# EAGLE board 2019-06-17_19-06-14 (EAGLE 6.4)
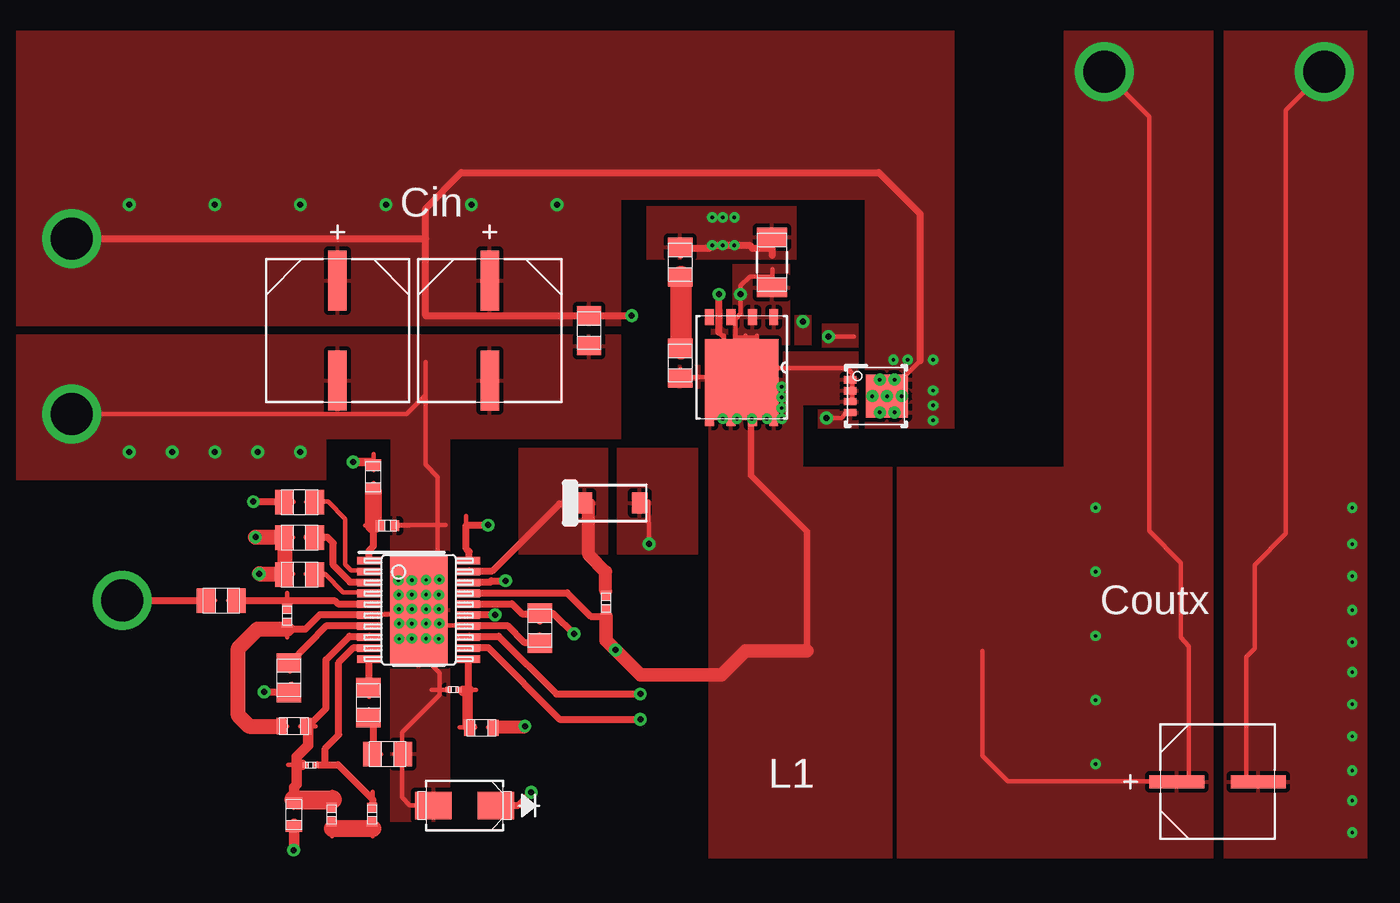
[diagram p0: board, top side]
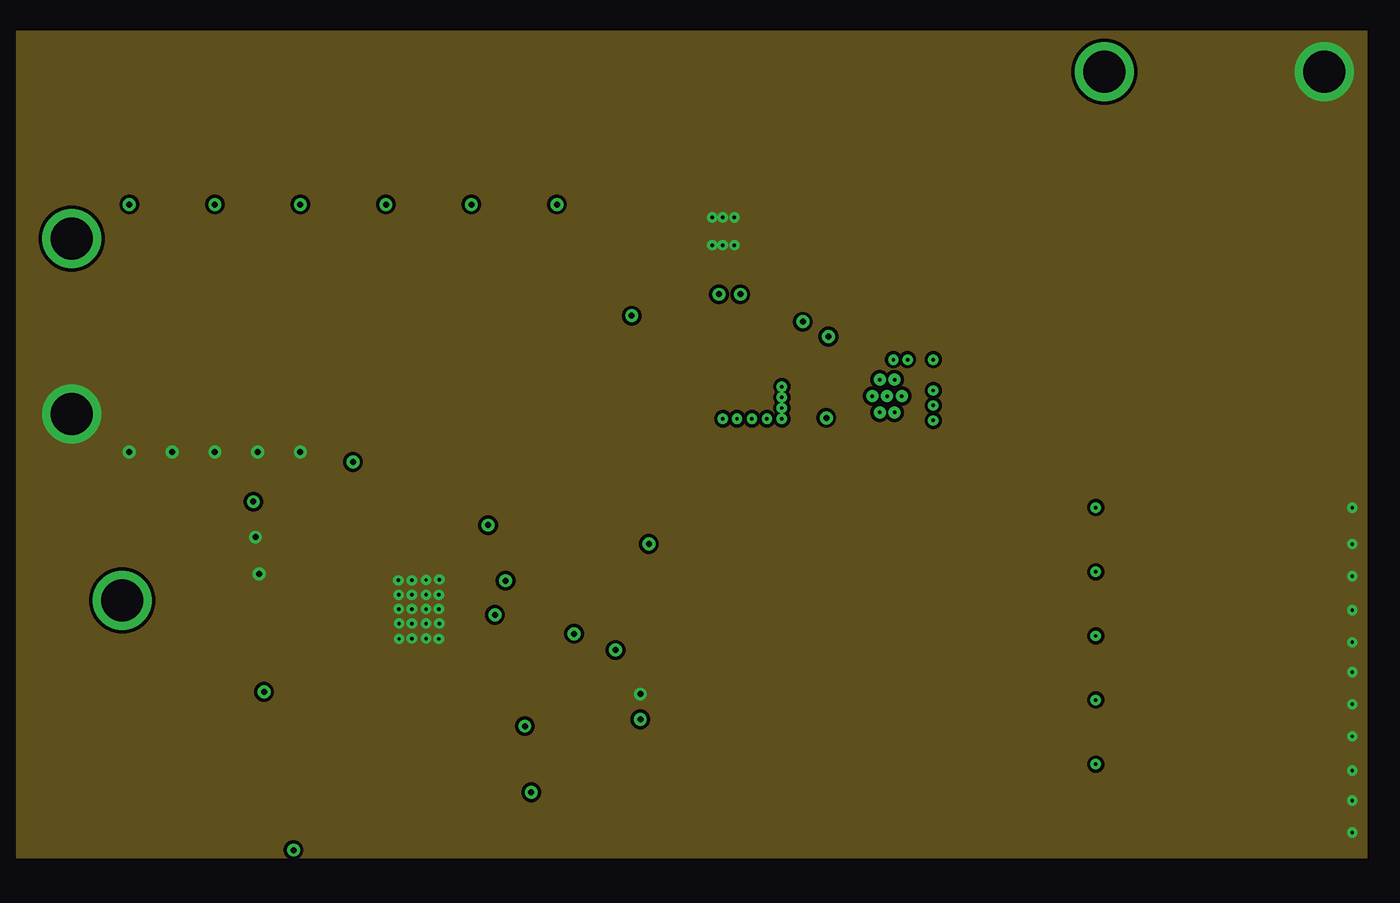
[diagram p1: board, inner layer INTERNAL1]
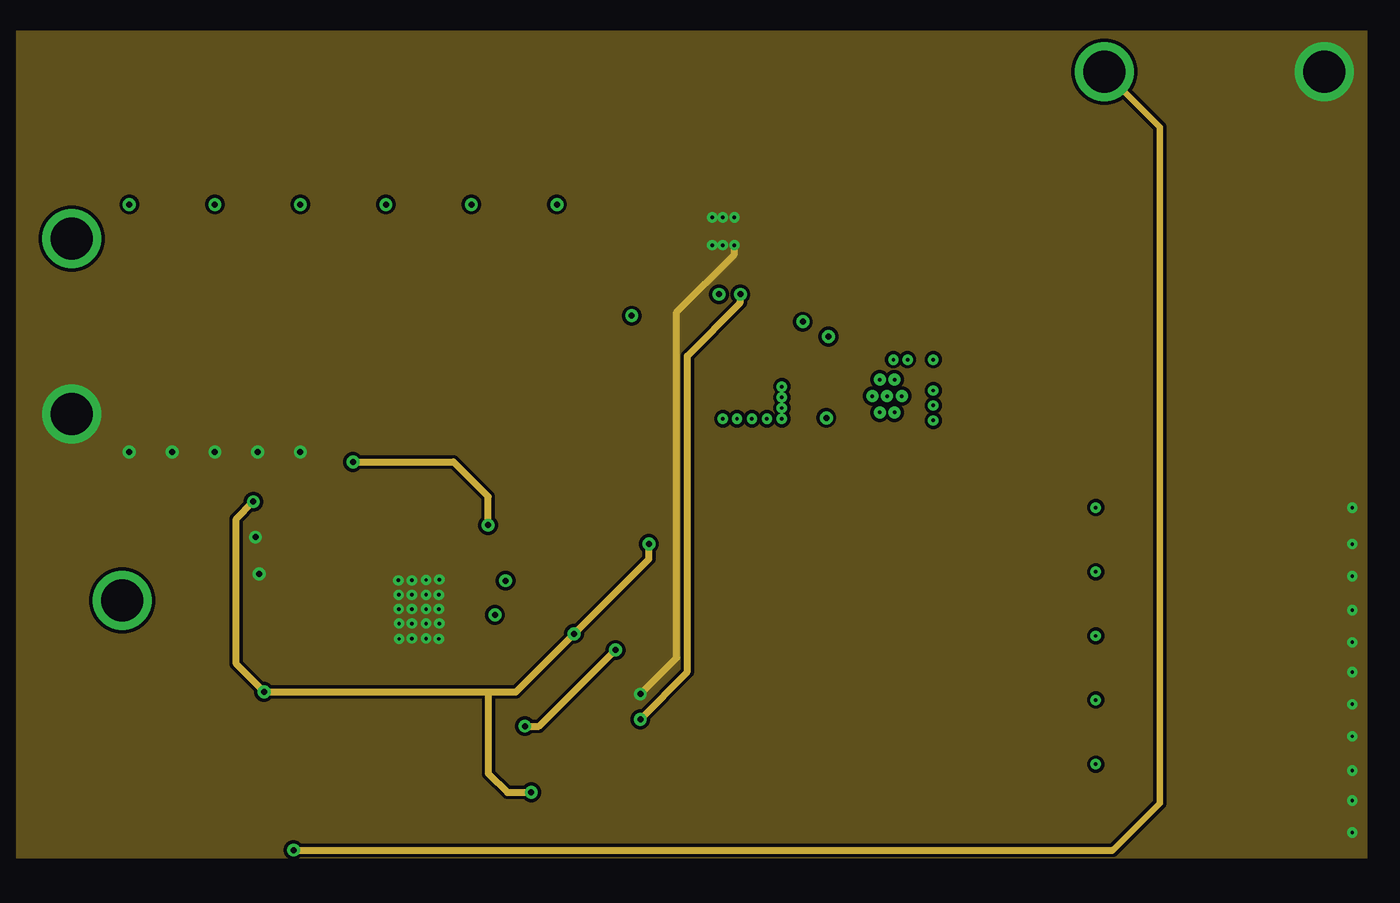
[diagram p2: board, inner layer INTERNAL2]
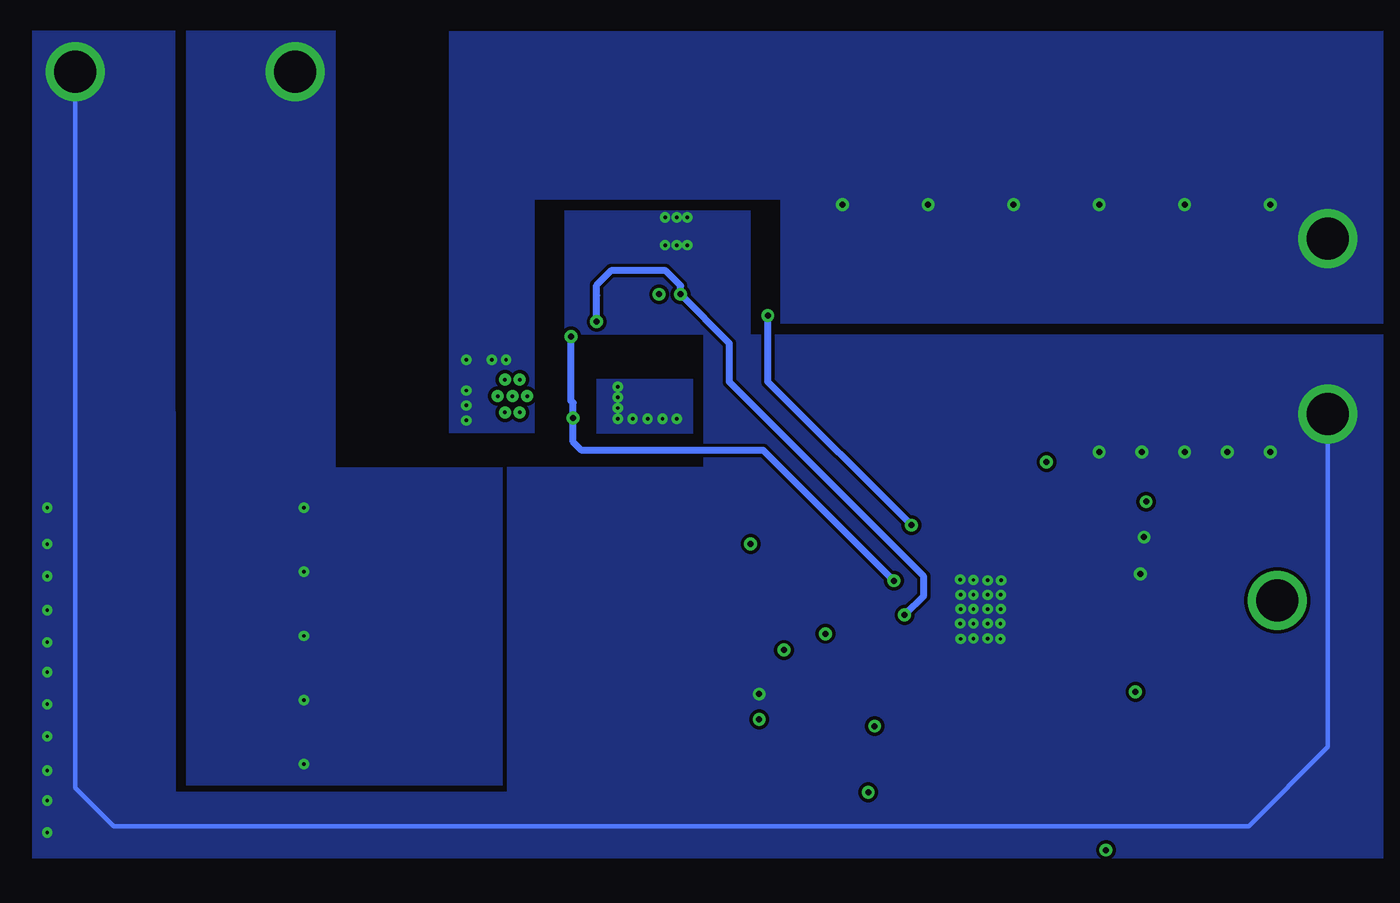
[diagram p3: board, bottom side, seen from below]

No outline drawn. Coordinates in mm, seen from the top.
Copper layers ((1*2)+(15*16)): TOP / INTERNAL1 / layer 15 / BOTTOM

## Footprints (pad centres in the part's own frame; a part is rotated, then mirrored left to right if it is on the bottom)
0402 = smd 0.559 x 0.61: 1 -0.419,0; 2 0.419,0
0805 = smd 1.118 x 1.448: 1 -0.902,0; 2 0.902,0
0201 = smd 0.356 x 0.33: 1 -0.292,0; 2 0.292,0
CAPSMT_62_E12 = smd 3.556 x 1.092: 1 -2.972,0; 2 2.972,0
SM_RADIAL_D8 = smd 3.251 x 0.762: 1 -2.426,0; 2 2.426,0
SOD-123 = smd 0.915 x 1.22: 1 -1.637,0; 2 1.637,0
SMA = smd 2.184 x 1.626: 1 -1.854,0; 2 1.854,0
TP-1502 = drill 0.813 round: 1 0,0
DQG0008A = smd 0.75 x 0.44: 1 -1.525,0.975; 2 -1.525,0.325; 3 -1.525,-0.325; 4 -1.525,-0.975; 5 1.525,-0.975; 6 1.525,-0.325; 7 1.525,0.325; 8 1.525,0.975 | smd 2.5 x 2.55: 9 0.65,0 | drill 0.203 round: V 0.226,0.975; V 1.102,0.975; V 1.102,-0.975; V 0.226,-0.975; V 0.664,0; V -0.212,0; V 1.54,0
PG-TDSON-8 = smd 0.965 x 0.533: 1 -2.997,1.905; 2 -2.997,0.635; 3 -2.997,-0.635; 4 -2.997,-1.905; 5 2.997,-1.905; 6 2.997,-0.635; 7 2.997,0.635; 8 2.997,1.905 | smd 4.805 x 4.36: 9 0.725,0
0603 = smd 0.66 x 0.965: 1 -0.699,0; 2 0.699,0
1206 = smd 1.118 x 1.803: 1 -1.499,0; 2 1.499,0
PWP0020A = smd 1.4 x 0.45: 1 -2.95,2.925; 2 -2.95,2.275; 3 -2.95,1.625; 4 -2.95,0.975; 5 -2.95,0.325; 6 -2.95,-0.325; 7 -2.95,-0.975; 8 -2.95,-1.625; 9 -2.95,-2.275; 10 -2.95,-2.925; 11 2.95,-2.925; 12 2.95,-2.275; 13 2.95,-1.625; 14 2.95,-0.975; 15 2.95,-0.325; 16 2.95,0.325; 17 2.95,0.975; 18 2.95,1.625; 19 2.95,2.275; 20 2.95,2.925 | smd 3.4 x 6.5: 21 0,0

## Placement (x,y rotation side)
Cboot  [0402]  61.09,40.97 270 top
Ccm  [0805]  48.11,31.98 0 top
Ccomp1  [0402]  47.19,28.37 270 top
Ccomp2  [0201]  43.54,31.32 180 top
Cin_1  [CAPSMT_62_E12]  54.18,57.12 270 top
Cin_2  [CAPSMT_62_E12]  45.14,57.12 270 top
Cinx  [0805]  60.07,57.12 270 top
Cout  [SM_RADIAL_D8]  97.41,30.33 0 top
Cramp  [0201]  52.02,35.79 180 top
Cres  [0805]  42.88,44.83 180 top
Csnub  [0805]  65.48,55.19 270 top
Css  [0805]  42.88,42.62 180 top
Csync  [0805]  38.23,41.07 0 top
Cvcc  [0805]  57.15,39.45 270 top
D1  [SOD-123]  61.44,46.89 0 top
D2  [SMA]  52.68,28.91 180 top
GND  [TP-1502]  103.73,72.47 0 top
GND1  [TP-1502]  29.34,52.12 0 top
M1  [DQG0008A]  77.11,53.24 0 top
M2  [PG-TDSON-8]  69.14,54.94 270 top
Rcm  [0805]  46.96,35.03 90 top
Rcomp  [0402]  44.78,28.37 90 top
RDemb  [0805]  42.88,46.94 0 top
Rfb1  [0603]  42.55,33.63 180 top
Rfb2  [0603]  42.55,28.37 90 top
Rramp  [0603]  53.67,33.53 180 top
Rsense  [1206]  70.94,61.19 90 top
Rsnub  [0805]  65.48,61.19 270 top
Rt  [0402]  42.14,40.18 270 top
Ruv1  [0402]  48.11,45.54 0 top
Ruv2  [0603]  47.24,48.44 270 top
Rvccdis  [0805]  42.24,36.5 90 top
U1  [PWP0020A]  49.96,40.54 0 top
VIN  [TP-1502]  29.34,62.53 0 top
VOUT  [TP-1502]  90.63,72.47 0 top
VSync  [TP-1502]  32.31,41.07 0 top

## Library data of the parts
Cboot = ultra-librarian; RefDes: Cboot; Type: GRM155R71A104KA01D
Ccm = ultra-librarian; RefDes: Ccm; Type: CC0805KRX7R9BB222
Ccomp1 = ultra-librarian; RefDes: Ccomp1; Type: CL05C821JB5NNNC
Ccomp2 = ultra-librarian; RefDes: Ccomp2; Type: GRM033R71C681KA01D
Cin_1 Cin_2 = ultra-librarian
Cinx = ultra-librarian; RefDes: Cinx; Type: C2012X7R2A104K125AA
Cout = ultra-librarian; RefDes: Cout; Type: EEE-FK1J220XP
Cramp = ultra-librarian; RefDes: Cramp; Type: GRM033R71E821KA01D
Cres = ultra-librarian; RefDes: Cres; Type: TMK212BJ474KD-T
Csnub = ultra-librarian; RefDes: Csnub; Type: CC0805KRX7R9BB153
Css = ultra-librarian; RefDes: Css; Type: CGA4F2C0G1H153J085AA
Csync = ultra-librarian; RefDes: Csync; Type: CC0805KRX7R9BB153
Cvcc = ultra-librarian; RefDes: Cvcc; Type: TMK212BJ474KD-T
D1 = ultra-librarian; RefDes: D1; Type: CDBW46-G
D2 = ultra-librarian; RefDes: D2; Type: B130L-13-F
GND = ultra-librarian; RefDes: GND; Type: TP-1502
GND1 = ultra-librarian; RefDes: GND1; Type: TP-1502
M1 = ultra-librarian; RefDes: M1; Type: CSD19537Q3
M2 = ultra-librarian; RefDes: M2; Type: BSC117N08NS5ATMA1
Rcm = ultra-librarian; RefDes: Rcm; Type: ERJ-6ENF3012V
Rcomp = ultra-librarian; RefDes: Rcomp; Type: CRCW040240K2FKED
RDemb = ultra-librarian; RefDes: RDemb; Type: ERJ-6ENF3012V
Rfb1 = ultra-librarian; RefDes: Rfb1; Type: RC0603FR-07910RL
Rfb2 = ultra-librarian; RefDes: Rfb2; Type: RC0603FR-0747KL
Rramp = ultra-librarian; RefDes: Rramp; Type: CRCW0603806KFKEA
Rsense = ultra-librarian; RefDes: Rsense; Type: CSR1206FK12L0
Rsnub = ultra-librarian; RefDes: Rsnub; Type: ERJ-6ENF3012V
Rt = ultra-librarian; RefDes: Rt; Type: CRCW04029K31FKED
Ruv1 = ultra-librarian; RefDes: Ruv1; Type: CRCW04021K30FKED
Ruv2 = ultra-librarian; RefDes: Ruv2; Type: CRCW060354K9FKEA
Rvccdis = ultra-librarian; RefDes: Rvccdis; Type: ERJ-6ENF3012V
U1 = ultra-librarian; RefDes: U1; Type: LM5117PMHX/NOPB
VIN = ultra-librarian; RefDes: VIN; Type: TP-1502
VOUT = ultra-librarian; RefDes: VOUT; Type: TP-1502
VSync = ultra-librarian; RefDes: VSync; Type: TP-1502

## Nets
0: Ccm.2 Cin_1.2 Cin_2.2 Cinx.2 Cout.2 Cramp.2 Cres.2 Css.2 Cvcc.2 D2.2 GND1.1 GND.1 Rfb1.2 Rsense.2 Rsnub.1 Rt.2 Ruv1.2 U1.6 U1.13 U1.14 U1.21
1: Cvcc.1 D1.2 D2.1 RDemb.1 RDemb.2 Rvccdis.1 U1.2 U1.16
2: Ccomp2.2 Rcomp.2 Rfb1.1 Rfb2.2 U1.8
3: Cboot.2 Csnub.2 M1.1 M1.2 M1.3 M2.5 M2.6 M2.7 M2.8 M2.9 Rramp.1 U1.17
4: Cboot.1 D1.1 U1.19
5: Cin_1.1 Cin_2.1 Cinx.1 M1.5 M1.6 M1.7 M1.8 M1.9 Ruv2.1 U1.20 VIN.1
6: Cramp.1 Rramp.2 U1.11
7: M2.1 M2.2 M2.3 Rsense.1 U1.12
8: Cout.1 Rfb2.1 VOUT.1
9: Csync.2 Rt.1 U1.5
10: Ruv1.1 Ruv2.2 U1.1
11: Ccomp1.1 Ccomp2.1 U1.9
12: Cres.1 U1.3
13: Css.1 U1.4
14: M1.4 U1.18
15: Ccomp1.2 Rcomp.1
17: Csync.1 VSync.1
18: Csnub.1 Rsnub.2
20: Rvccdis.2 U1.7
27: Rcm.2 U1.10
35: Ccm.1 Rcm.1
S$22netdata: M2.4 U1.15

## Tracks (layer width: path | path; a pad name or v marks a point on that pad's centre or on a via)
0  (via drill 0.2 pad 0.61, 0.36 pad 0.76, 2.49 pad 3.48)
  TOP 0.254: 51.08,45.57 51.56,45.57 | 51.21,35.79 51.69,35.79 | 51.21,35.79 51.21,36.8 49.99,38.02 49.99,40.59 | 48.51,31.98 48.97,31.98 | 52.96,39.6 50.95,39.6 50.8,39.75 50.8,40.59 49.99,40.59 | 51.08,45.57 51.08,43.74 49.99,42.65 49.99,40.59 | 48.51,45.57 51.08,45.57 | 47.02,40.26 48.39,40.26 48.72,40.59 49.99,40.59 | 51.08,45.57 51.08,48.44 50.37,49.17 50.37,53.31 | 51.21,35.79 51.21,35.48 48.97,33.25 48.97,31.98 | 50.7,28.93 49.43,28.93 48.97,29.39 48.97,31.98 | v29.34,52.17 49.23,52.17 50.37,53.31 | 50.37,53.31 50.37,55.27 | v103.76,72.52 101.47,70.23 101.47,45.09 99.62,43.2 99.62,40.89 99.62,38.25 99.11,37.74 99.11,30.35 | 49.86,28.91 51.49,28.91 | 70.98,61.54 70.98,62.48 | 65.52,61.54 65.52,62.48 | 51.07,44.98 51.07,46.13 | 48.49,31.97 49.43,31.97 | 41.2,33.62 42.14,33.62 | 57.14,38.12 57.14,39.06 | 41.55,44.84 42.49,44.84 | 41.55,42.66 42.49,42.66 | 42.15,38.91 42.15,39.85 | 48.49,45.55 49.43,45.55 | 50.72,35.78 51.66,35.78
  TOP 0.406: 70.97,61.59 70.97,62.03 69.77,62.03 69.62,62.2 v68.71,62.2 v68.02,62.2 v67.39,62.2 67.21,62.03 65.53,62.03 65.53,61.59 | 52.96,39.6 55.22,39.6 56.21,38.61 57.15,38.61 | 47.02,40.26 44.09,40.26 43.23,39.4 42.16,39.4 | v63.12,35.53 58.14,35.53 54.71,38.96 52.96,38.96
  TOP 0.889: 42.16,39.4 40.39,39.4 39.24,38.25 39.24,34.27 39.88,33.63 41.68,33.63 | v40.49,42.67 42.04,42.67 42.04,44.86 v40.26,44.86
  INTERNAL2 0.406: v63.12,35.53 65.28,37.69 65.28,58.22 68.71,61.65 v68.71,62.2
  BOTTOM 0.254: v103.76,72.52 103.76,29.97 101.47,27.69 34.04,27.69 29.34,32.38 v29.34,52.17
  other vias: 105.41,30.99 105.41,34.92 105.41,38.61 105.41,42.55 105.41,46.61 105.41,29.21 105.41,27.3 105.41,44.45 105.41,40.51 105.41,36.83 105.41,33.02 42.93,49.91 40.39,49.91 37.85,49.91 35.31,49.91 32.77,49.91 51.18,39.73 48.79,39.73 50.39,39.73 49.56,39.73 67.39,63.86 68.02,63.86 68.71,63.86 48.79,38.81 49.56,38.84 50.39,38.84 51.16,38.81 49.56,42.29 48.74,42.29 50.39,42.32 51.18,42.34 51.16,41.43 50.39,41.43 49.56,41.43 48.77,41.43 50.39,40.59 49.56,40.59 48.77,40.59 51.16,40.59
  pour TOP (rank 6): 97.79,74.93 106.3,74.93 106.3,25.78 97.79,25.78
  pour TOP (rank 6): 63.5,64.52 72.39,64.52 72.39,61.34 63.5,61.34
  pour TOP: 51.82,27.94 48.26,27.94 48.26,40.11 46.1,40.11 46.1,40.44 48.26,40.44 48.29,50.67 44.45,50.67 44.45,48.26 26.04,48.26 26.04,56.9 61.98,56.9 61.98,50.67 51.82,50.67
  pour BOTTOM (rank 6): 26.04,56.9 63.63,56.9 63.63,64.26 74.68,64.26 74.68,56.9 66.42,56.9 66.42,49.02 78.11,49.02 78.11,29.72 97.79,29.72 97.82,74.93 106.3,74.93 106.3,25.78 26.04,25.78
  pour INTERNAL1 (rank 5): 26.04,74.93 106.3,74.93 106.3,25.78 26.04,25.78
  pour INTERNAL2 (rank 5): 26.04,74.93 26.04,25.78 106.3,25.78 106.3,74.93
1  (via drill 0.36 pad 0.76)
  TOP 0.254: v63.63,44.45 63.63,45.67 63.6,45.72 63.6,46.99 | 43.31,46.97 43.76,46.97 44.58,46.97 45.59,45.95 45.59,43.23 45.95,42.88 47.04,42.88 | 53.87,28.91 55.5,28.91 | 41.58,46.95 42.52,46.95 | 43.28,46.95 44.22,46.95 | 57.14,39.83 57.14,40.77 | 42.28,35.18 42.28,36.12
  TOP 0.406: 42.06,46.97 42.42,46.97 | 42.06,46.97 | v40.13,46.97 42.06,46.97 | 57.15,39.88 57.15,40.31 | 42.42,36.07 42.42,35.81 42.29,35.66 v40.77,35.66 | v56.64,29.69 55.88,28.93 54.69,28.93 | v40.77,35.66 | v59.18,39.12 57.96,40.31 57.15,40.31 | 57.15,40.31 56.08,40.31 55.5,40.89 52.96,40.89
  INTERNAL2 0.406: v63.63,44.45 63.63,43.56 v59.18,39.12 55.73,35.66 54.1,35.66 | 54.1,35.66 v40.77,35.66 39.12,37.31 39.12,45.95 v40.13,46.97 | 54.1,35.66 54.1,30.81 55.22,29.69 v56.64,29.69
  pour TOP (rank 3): 61.72,50.16 61.72,43.81 66.55,43.81 66.55,50.16
2
  TOP 0.254: 42.53,28.78 42.53,29.72 | 42.9,33.62 43.84,33.62 | 42.22,31.33 43.16,31.33 | 44.82,28.78 44.82,29.72
  TOP 0.406: 43.38,33.63 44.45,34.67 44.45,37.57 45.85,38.96 47.02,38.96
  TOP 0.635: 42.7,31.34 42.7,30.18 42.55,30 42.55,29.26 | 42.7,31.34 42.7,31.8 43.38,32.49 43.38,33.63 | 42.7,31.34 43.03,31.34
  TOP 1.143: 42.55,29.26 44.83,29.26
3  (via drill 0.2 pad 0.61, 0.36 pad 0.76)
  TOP 0.254: 69.7,53.19 70.05,53.52 70.05,53.7 69.39,53.7 68.76,53.7 | 75.72,52.88 75.72,53.54 | 75.72,53.54 | 75.72,53.54 75.72,54.18 75.72,54.59 75.41,54.89 69.06,54.89 | 69.06,54.89 68.76,54.56 68.76,53.7 | 68.1,53.7 68.76,53.7 | 69.06,54.89 67.61,54.89 67.08,54.38 65.53,54.38 | 69.7,51.84 v69.75,51.89 | 67.79,57.02 67.79,57 68.1,56.72 | 75.59,52.87 75.84,52.87 | 75.59,53.53 75.84,53.53 | 75.59,54.17 75.84,54.17 | 69.06,54.08 69.06,55.68 | 70.04,53.67 70.04,53.72 | 69.38,53.67 69.38,53.72 | 68.75,53.67 68.75,53.72 | 68.08,53.67 68.08,53.72 | 68.08,56.54 68.08,56.84 | 54.08,33.57 55.02,33.57 | 65.52,53.9 65.52,54.84 | 61.07,39.67 61.07,40.62
  TOP 0.381: 69.7,51.84 69.7,51.08 69.7,48.51 73.03,45.19 73.03,38.1
  TOP 0.406: 69.7,51.89 69.7,53.19 | 61.09,40.16 60.17,40.16 58.78,41.55 52.96,41.55 | 67.79,57.02 v67.79,59.28 | 52.96,40.26 54.43,40.26 v54.48,40.23
  TOP 0.762: v56.26,33.63 56.21,33.58 54.56,33.58
  TOP 0.813: 61.09,40.16 61.09,38.71 63.12,36.68 67.94,36.68 69.37,38.1 73.03,38.1
  INTERNAL2 0.406: v56.26,33.63 57.1,33.63 v61.65,38.15
  BOTTOM 0.406: v72.77,57.66 72.77,59.23 72.77,59.82 71.93,60.68 68.68,60.68 67.79,59.79 v67.79,59.28 64.9,56.36 64.9,54.08 53.34,42.52 53.34,41.38 v54.48,40.23
  other vias: 68.02,51.89 71.53,51.89 71.53,53.16 71.53,53.8 70.64,51.89 68.86,51.89 71.53,52.53
  pour TOP (rank 2): 76.07,55.88 76.07,52.7 72.77,52.7 72.77,49.02 78.11,49.02 78.11,25.78 67.18,25.78 67.18,53.7 64.77,53.7 64.77,55.09 67.18,55.09 67.18,55.88
  pour TOP (rank 4): 73.28,56.26 72.26,56.26 72.26,58.04 73.28,58.04
  pour TOP (rank 4): 68.33,56.26 68.33,58.42 67.31,58.42 67.31,56.26
  pour BOTTOM: 67.06,54.25 67.06,51 72.77,51 72.77,54.25
4
  TOP 0.254: 61.07,41.38 61.07,42.32
  TOP 0.406: 60.05,46.84 58.32,46.84 54.33,42.85 52.96,42.85
  TOP 0.762: 60.05,46.84 60.05,43.81 61.06,42.8 61.06,41.66
  pour TOP (rank 5): 61.21,50.16 61.21,43.81 55.88,43.81 55.88,49.53 55.88,50.16
5  (via drill 0.2 pad 0.61, 0.36 pad 0.76, 2.49 pad 3.48)
  TOP 0.254: 79.76,55.35 78.59,54.18 78.59,53.54 | 78.59,52.25 78.59,53.54 | 78.59,53.54 77.93,53.54 77.62,53.21 77.17,53.21 | 77.04,53.2 77.29,53.2 | 78.46,54.17 78.72,54.17 | 78.46,53.53 78.72,53.53 | 78.46,52.87 78.72,52.87 | 78.46,52.23 78.72,52.23 | 47.28,48.84 47.28,49.78 | 52.77,44.98 52.77,46.13
  TOP 0.406: 79.76,55.35 79.76,64.06 77.29,66.52 52.48,66.52 50.37,64.39 50.37,62.59 | 52.96,43.51 52.96,43.99 52.78,44.17 52.78,45.57 v54.08,45.57 | v29.34,62.59 50.37,62.59 | 50.37,62.59 50.37,58.01 v62.61,58.01
  TOP 0.508: 47.27,49.02 47.27,49.3 | v46.05,49.33 47.24,49.33
  INTERNAL2 0.406: v46.05,49.33 52.02,49.33 54.08,47.27 v54.08,45.57
  BOTTOM 0.406: v54.08,45.57 62.61,54.08 v62.61,58.01
  other vias: 58.17,64.62 53.09,64.62 48.01,64.62 42.93,64.62 37.85,64.62 32.77,64.62 78.16,55.4 80.52,55.4 80.52,53.57 80.52,52.68 80.52,51.79 78.99,55.4
  pour TOP (rank 3): 26.04,74.93 81.79,74.93 81.79,51.31 76.45,51.31 76.45,64.9 61.98,64.9 61.98,57.4 26.04,57.4
  pour BOTTOM: 76.45,51.05 81.53,51.05 81.53,74.9 26.04,74.93 26.04,57.53 61.85,57.53 61.85,64.9 76.45,64.9
6
  TOP 0.254: 52.38,33.57 53.31,33.57 | 52.43,35.78 53.37,35.78
  TOP 0.406: 52.91,35.79 52.91,37.59 52.96,37.64
  TOP 0.635: 52.58,35.74 52.86,35.74 | 52.86,35.74 52.91,35.79 | 52.86,35.74 52.86,33.58 53.09,33.58
7  (via drill 0.36 pad 0.76)
  TOP 0.254: 70.97,60.33 69.62,60.33 69.06,59.79 v69.06,59.28 69.06,58.14 68.76,57.81 68.76,56.72 69.39,56.72 70.05,56.72 | 68.75,56.54 68.75,56.84 | 69.38,56.54 69.38,56.84 | 70.04,56.54 70.04,56.84 | 70.98,59.84 70.98,60.78
  TOP 0.406: v63.12,34.04 58.32,34.04 54.08,38.3 52.96,38.3
  INTERNAL2 0.406: v63.12,34.04 65.91,36.85 65.91,55.63 69.06,58.8 v69.06,59.28
  pour TOP (rank 2): 68.58,56.26 72.01,56.26 72.01,61.09 68.58,61.09
8  (via drill 0.2 pad 0.61, 0.36 pad 0.76, 2.49 pad 3.48)
  TOP 0.254: v90.68,72.52 93.34,69.85 93.34,45.21 95.22,43.33 95.22,40.89 95.22,38.89 95.71,38.38 95.71,30.35 84.96,30.35 83.44,31.88 83.44,38.1 | 42.53,27.08 42.53,28.02
  TOP 0.635: 42.55,27.81 42.55,27.79 42.55,27.56 42.55,26.26
  INTERNAL2 0.381: 91.19,26.26 93.98,29.06 93.98,69.22 v90.68,72.52
  INTERNAL2 0.406: v42.52,26.26 91.19,26.26
  other vias: 90.17,46.61 90.17,42.8 90.17,31.37 90.17,35.18 90.17,38.99
  pour TOP (rank 2): 78.36,25.78 97.16,25.78 97.16,74.93 88.27,74.93 88.27,49.02 78.36,49.02
  pour BOTTOM: 78.36,30.1 97.16,30.1 97.16,74.93 88.27,74.93 88.27,49.02 78.36,49
9
  TOP 0.254: 38.63,41.08 39.57,41.08 | 42.15,40.62 42.15,41.55
  TOP 0.406: 39.12,41.1 42.14,41.1 42.16,41.1 44.96,41.1 45.16,40.89 47.02,40.89
10
  TOP 0.254: 47.28,47.14 47.28,48.08 | 46.79,45.55 47.73,45.55
  TOP 0.406: 47.02,43.51 47.02,44.07 47.27,44.32 47.27,45.57
  TOP 1.016: 47.27,45.57 47.27,47.6
11
  TOP 0.254: 43.92,31.33 44.86,31.33 | 47.23,28.78 47.23,29.72
  TOP 0.406: 47.24,28.83 47.24,29.26 45.16,31.34 44.4,31.34 | 43.94,31.34 44.4,31.34 | 44.4,31.34 44.4,32.31 45.21,33.12 45.21,37.41 46.1,38.3 47.02,38.3
12
  TOP 0.254: 47.02,42.22 47.04,42.22 | 43.26,44.84 44.2,44.84
  TOP 0.406: 43.31,44.86 43.74,44.86 44.53,44.86 44.88,44.5 44.88,43.2 45.87,42.19 47.02,42.19
13
  TOP 0.254: 43.23,42.67 | 43.23,42.67 43.74,42.67 44.4,42.67 45.47,41.58 47.04,41.58 | 43.26,42.66 44.2,42.66
14  (via drill 0.36 pad 0.76)
  TOP 0.254: 75.72,52.25 75.36,52.25 75.06,51.94 v74.17,51.94 | v74.3,56.77 75.82,56.77 | 75.59,52.23 75.84,52.23
  TOP 0.406: 52.96,42.19 54.2,42.19 54.25,42.27 v55.12,42.27
  BOTTOM 0.406: v74.3,56.77 74.3,52.96 74.17,52.83 v74.17,51.94 74.17,50.52 73.66,50.01 62.87,50.01 v55.12,42.27
  pour TOP (rank 3): 76.07,52.45 73.66,52.45 73.66,51.31 76.07,51.31
  pour TOP (rank 4): 76.07,56.13 76.07,57.53 73.91,57.53 73.91,56.13
15
  TOP 0.254: 47.23,27.08 47.23,28.02 | 44.82,27.08 44.82,28.02
  TOP 1.016: 44.83,27.56 47.24,27.56
17  (via drill 2.49 pad 3.48)
  TOP 0.254: 36.93,41.08 37.87,41.08
  TOP 0.406: 37.41,41.1 37.39,41.1 v32.33,41.1
18
  TOP 0.254: 65.52,59.84 65.52,60.78 | 65.52,55.6 65.52,56.54
  TOP 1.27: 65.53,56.06 65.53,60.33
20
  TOP 0.254: 42.28,36.88 42.28,37.82
  TOP 0.406: 42.29,36.96 42.29,37.36 44.5,39.6 47.02,39.6
27
  TOP 0.254: 47,35.38 47,36.32
  TOP 0.406: 46.99,35.48 47.02,35.48 47.02,35.87 47.02,37.64
35
  TOP 0.254: 47,33.68 47,34.62 | 46.79,31.97 47.73,31.97
  TOP 0.406: 46.99,34.54 47.02,34.52 47.02,34.16 47.27,33.91 47.27,31.98 47.62,31.98

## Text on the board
ASSYNOTES: Cin | Coutx | L1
